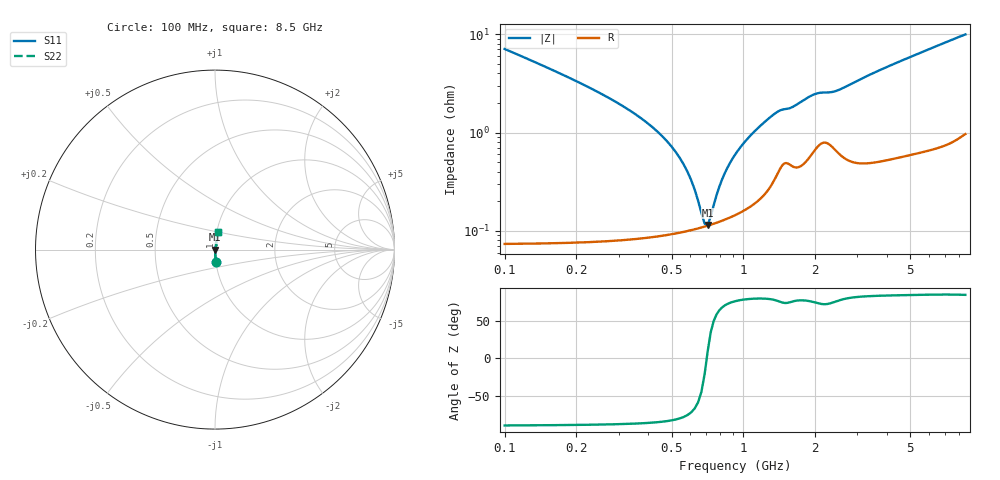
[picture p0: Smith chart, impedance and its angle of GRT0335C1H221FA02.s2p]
!Murata Part Number: GRT0335C1H221FA02
!These Parameters are Measured in Series Mode Connection
!Data Generated on Jun 19, 2026
!  o--ll--o
!Port1  Port2
!  o------o
!Operation Temp=25[degC], DC Bias Voltage=0[V]
!Freq. Start=100[MHz] Stop=9[GHz] 401[Steps]
# Hz S RI R 50
!Freq.(Hz) S11(Real) S11(Imag) S21(Real) S21(Imag) S12(Real) S12(Imag) S22(Real) S22(Imag)
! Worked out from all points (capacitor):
!   401 points, 100 MHz to 8.5 GHz, reference 50 ohm
!   read as one part in series: C = 220 pF near 142 MHz
!   lowest |Z| = 115 mohm at 709 MHz (marker M1)
!   series resonance near 702.2 MHz, so ESL is about 230 pH
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1e8  0.00572 -0.0704  0.9943 0.0704  0.9943 0.0704  0.00572 -0.0704
2.26e8  0.00159 -0.0286  0.9984 0.0286  0.9984 0.0286  0.00159 -0.0286
4.99e8  0.000974 -0.00718  0.999 0.00718  0.999 0.00718  0.000974 -0.00718
5.83e8  0.00101 -0.00386  0.999 0.00386  0.999 0.00386  0.00101 -0.00386
6.67e8  0.00108 -0.00106  0.9989 0.00106  0.9989 0.00106  0.00108 -0.00106
6.88e8  0.0011 -0.000422  0.9989 0.000422  0.9989 0.000422  0.0011 -0.000422
7.09e8  0.00113 0.0002  0.9989 -0.0002  0.9989 -0.0002  0.00113 0.0002
7.3e8  0.00115 0.000805  0.9988 -0.000805  0.9988 -0.000805  0.00115 0.000805
8.14e8  0.00128 0.00308  0.9987 -0.00308  0.9987 -0.00308  0.00128 0.00308
8.56e8  0.00135 0.00415  0.9987 -0.00415  0.9987 -0.00415  0.00135 0.00415
9.82e8  0.00161 0.00715  0.9984 -0.00715  0.9984 -0.00715  0.00161 0.00715
1.108e9  0.00197 0.00996  0.998 -0.00996  0.998 -0.00996  0.00197 0.00996
1.255e9  0.00268 0.0131  0.9973 -0.0131  0.9973 -0.0131  0.00268 0.0131
1.381e9  0.00393 0.0156  0.9961 -0.0156  0.9961 -0.0156  0.00393 0.0156
1.507e9  0.00515 0.0165  0.9949 -0.0165  0.9949 -0.0165  0.00515 0.0165
1.99e9  0.00712 0.0234  0.9929 -0.0234  0.9929 -0.0234  0.00712 0.0234
2.41e9  0.00732 0.025  0.9927 -0.025  0.9927 -0.025  0.00732 0.025
2.914e9  0.00594 0.0318  0.9941 -0.0318  0.9941 -0.0318  0.00594 0.0318
4.3e9  0.00786 0.0494  0.9921 -0.0494  0.9921 -0.0494  0.00786 0.0494
5.707e9  0.0107 0.0657  0.9893 -0.0657  0.9893 -0.0657  0.0107 0.0657
7.114e9  0.0142 0.0817  0.9858 -0.0817  0.9858 -0.0817  0.0142 0.0817
8.5e9  0.019 0.0962  0.981 -0.0962  0.981 -0.0962  0.019 0.0962
